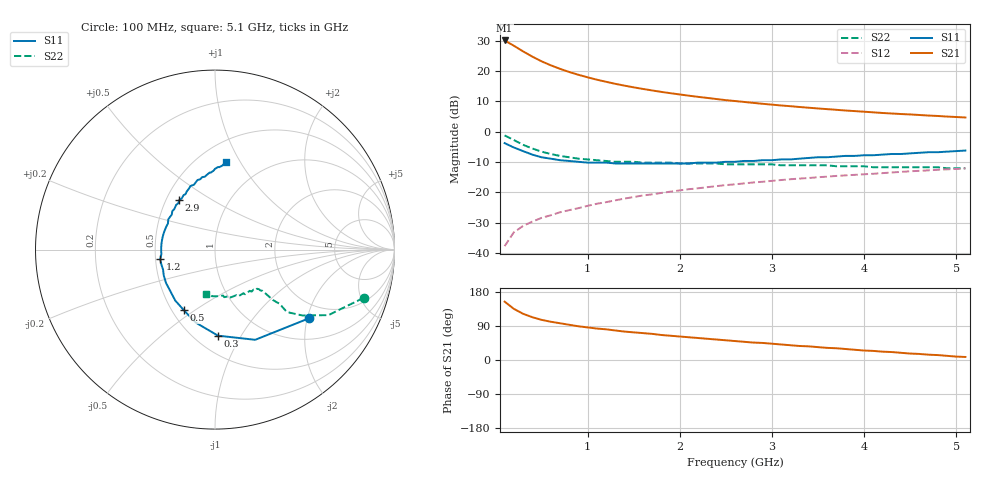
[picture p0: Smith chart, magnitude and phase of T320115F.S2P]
!AT-32011
!S PARAMETERS at Vce=5  V  Ic=15mA.  LAST UPDATED 01-05-95
# ghz s ma r 50
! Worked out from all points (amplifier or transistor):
!   51 points, 100 MHz to 5.1 GHz, reference 50 ohm
!   highest |S21| = 30.1 dB at 100 MHz (marker M1)
!   |S21| within 3 dB of that: start of sweep to 267.9 MHz
!   unconditionally stable (mu >= 1): 1.183 GHz to 4.928 GHz
!   at 900 MHz: K = 0.94, MSG = 22.0 dB, |S12| = -25.2 dB
!   at 2.6 GHz: K = 1.08, MAG = 12.0 dB, |S12| = -17.3 dB
!   at 5.1 GHz: K = 0.98, MSG = 8.4 dB, |S12| = -12.1 dB
!   S11 on the Smith chart (normalised r, x): 100 MHz: 1.56, -2.06; 300 MHz: 0.64, -0.80; 500 MHz: 0.57, -0.45; 1.2 GHz: 0.53, -0.06; 2.9 GHz: 0.58, +0.36; 5.1 GHz: 0.68, +0.87
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0.1  0.65 -36.0  31.99 154.0  0.013 74.0  0.87 -18.0
0.2  0.55 -66.0  26.2 135.0  0.022 65.0  0.73 -30.0
0.3  0.48 -88.0  21.14 122.0  0.028 60.0  0.61 -37.0
0.4  0.42 -105.0  17.35 113.0  0.033 59.0  0.53 -41.0
0.5  0.38 -117.0  14.51 106.0  0.038 59.0  0.47 -40.0
0.6  0.36 -128.0  12.48 101.0  0.042 59.0  0.43 -41.0
0.7  0.34 -137.0  10.91 97.0  0.047 60.0  0.4 -41.0
0.8  0.33 -146.0  9.68 93.0  0.051 60.0  0.38 -41.0
0.9  0.32 -153.0  8.7 89.0  0.055 61.0  0.36 -41.0
1  0.31 -159.0  7.9 86.0  0.06 61.0  0.35 -41.0
1.1  0.31 -164.0  7.22 83.0  0.065 61.0  0.34 -42.0
1.2  0.31 -170.0  6.67 81.0  0.069 61.0  0.33 -42.0
1.4  0.3 -180.0  5.76 75.0  0.079 61.0  0.32 -44.0
1.6  0.3 171.0  5.08 71.0  0.089 60.0  0.31 -46.0
1.8  0.3 163.0  4.54 66.0  0.098 59.0  0.31 -48.0
2.2  0.31 147.0  3.76 58.0  0.117 57.0  0.3 -53.0
2.6  0.32 135.0  3.21 50.0  0.136 54.0  0.29 -58.0
2.9  0.34 126.0  2.89 45.0  0.15 51.0  0.29 -63.0
3.5  0.38 111.0  2.42 34.0  0.178 47.0  0.28 -71.0
4  0.41 100.0  2.14 25.0  0.199 42.0  0.27 -79.0
4.3  0.43 94.0  2 21.0  0.213 40.0  0.26 -83.0
5.1  0.49 83.0  1.72 8.0  0.248 32.0  0.25 -101.0
